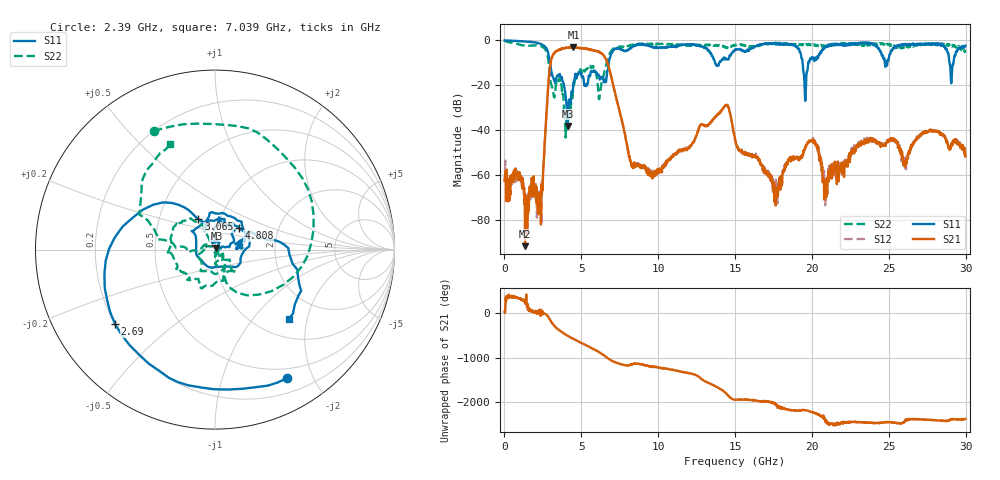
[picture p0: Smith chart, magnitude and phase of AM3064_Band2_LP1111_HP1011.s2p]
# Hz S DB R 50.0
!freq dBS11 angS11 dBS21 angS21 dBS12 angS12 dBS22 angS22
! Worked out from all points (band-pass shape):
!   1600 points, 10 MHz to 29.98 GHz, reference 50 ohm
!   highest |S21| = -3.03 dB at 4.49 GHz (marker M1); lowest = -91.6 dB at 1.341 GHz (marker M2)
!   |S21| within 3 dB of the highest: 3.201 GHz to 6.352 GHz (3.151 GHz wide, 66 % of centre)
!   lowest |S11| = -38.0 dB at 4.115 GHz (marker M3), VSWR 1.03, Z = 50.8 + j0.97 ohm
!   |S11| at or under -10 dB: 2.955 GHz to 6.784 GHz (3.829 GHz wide, 78.6 % of centre); 19.39 GHz to 19.76 GHz (368.2 MHz wide, 1.88 % of centre); 28.95 GHz to 29.2 GHz (254.4 MHz wide, 0.875 % of centre)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
!   |S22| runs from -43.2 to -0.1 dB; largest |S21 - S12| = 0.025
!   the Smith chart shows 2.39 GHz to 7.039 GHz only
!   S11 on the Smith chart (normalised r, x): 2.39 GHz: 0.37, -1.64; 2.69 GHz: 0.20, -0.32; 3.065 GHz: 0.79, +0.28; 4.808 GHz: 1.26, +0.31; 7.039 GHz: 1.38, -1.56
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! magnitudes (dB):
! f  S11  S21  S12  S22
! 10 MHz  0.0  -62.3  -60.3  -0.1
! 1.341 GHz  -0.6  -91.6  -70.4  -2.4
! 2.39 GHz  -1.7  -75.6  -72.4  -2.6
! 2.69 GHz  -3.2  -37.4  -37.2  -4.4
! 3.065 GHz  -14.3  -8.0  -8.0  -20.0
! 4.115 GHz  -38.0  -3.3  -3.1  -36.9
! 4.49 GHz  -18.7  -3.0  -3.2  -20.0
! 4.808 GHz  -15.0  -3.3  -3.2  -14.8
! 5.015 GHz  -15.7  -3.4  -3.5  -14.0
! 6.214 GHz  -17.2  -5.4  -5.2  -23.5
! 7.039 GHz  -5.0  -18.8  -18.8  -3.9
! 8.257 GHz  -3.1  -56.0  -55.9  -2.0
! 10 GHz  -3.3  -59.0  -58.8  -1.7
! 14.37 GHz  -8.5  -28.9  -28.8  -3.2
! 15 GHz  -4.1  -44.4  -44.2  -2.1
! 17.67 GHz  -1.9  -67.4  -63.8  -1.3
! 19.03 GHz  -2.9  -51.7  -52.7  -1.9
! 19.56 GHz  -26.9  -47.5  -47.6  -1.8
! 19.99 GHz  -7.5  -44.5  -44.9  -1.6
! 20.85 GHz  -3.2  -67.6  -62.6  -2.4
! 25 GHz  -8.5  -44.1  -45.5  -1.6
! 29.98 GHz  -2.4  -51.7  -51.1  -4.4
